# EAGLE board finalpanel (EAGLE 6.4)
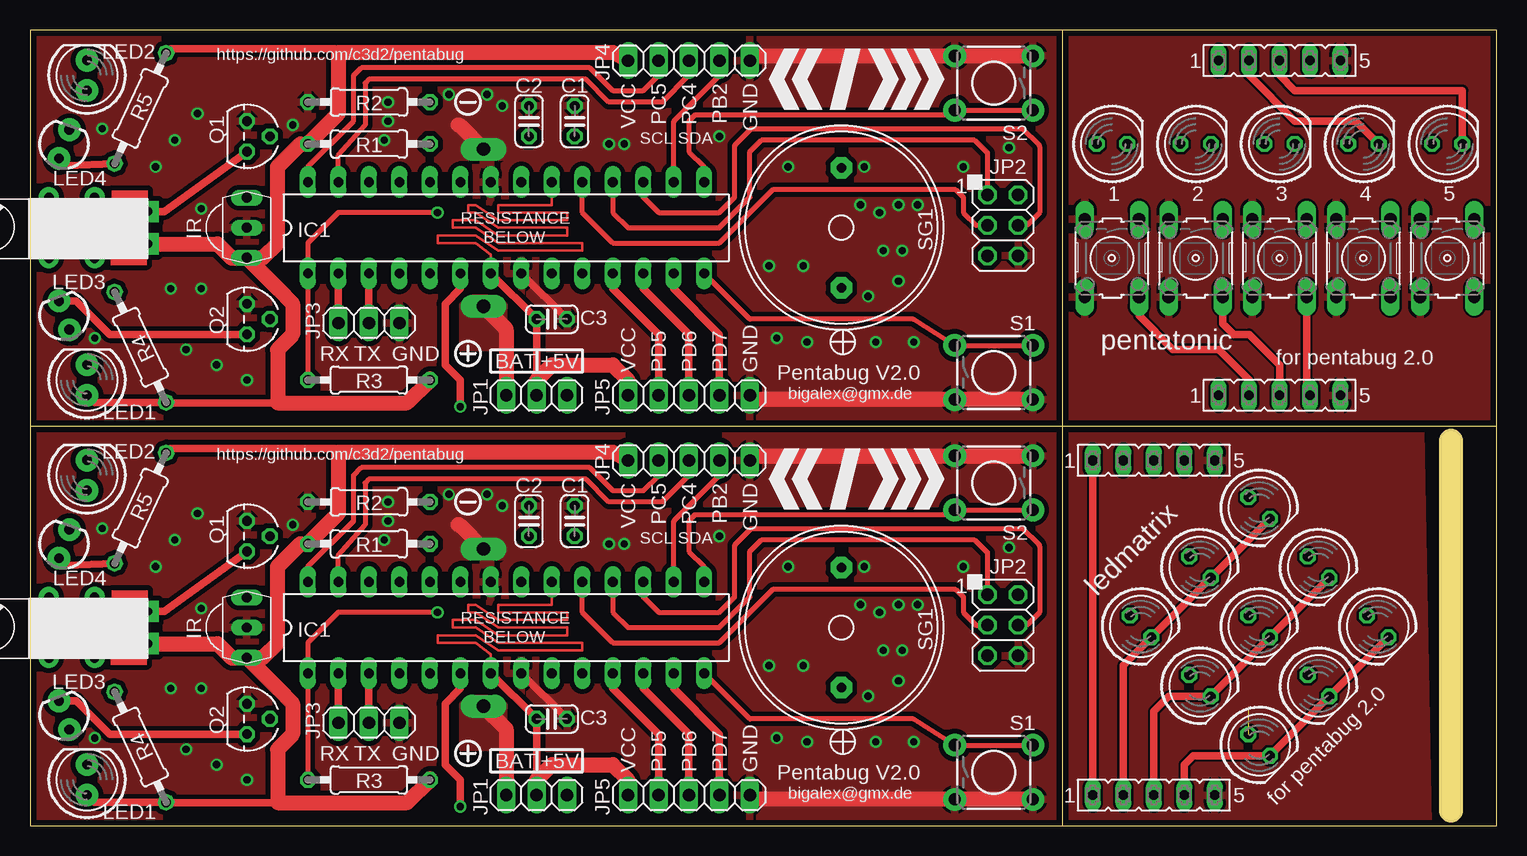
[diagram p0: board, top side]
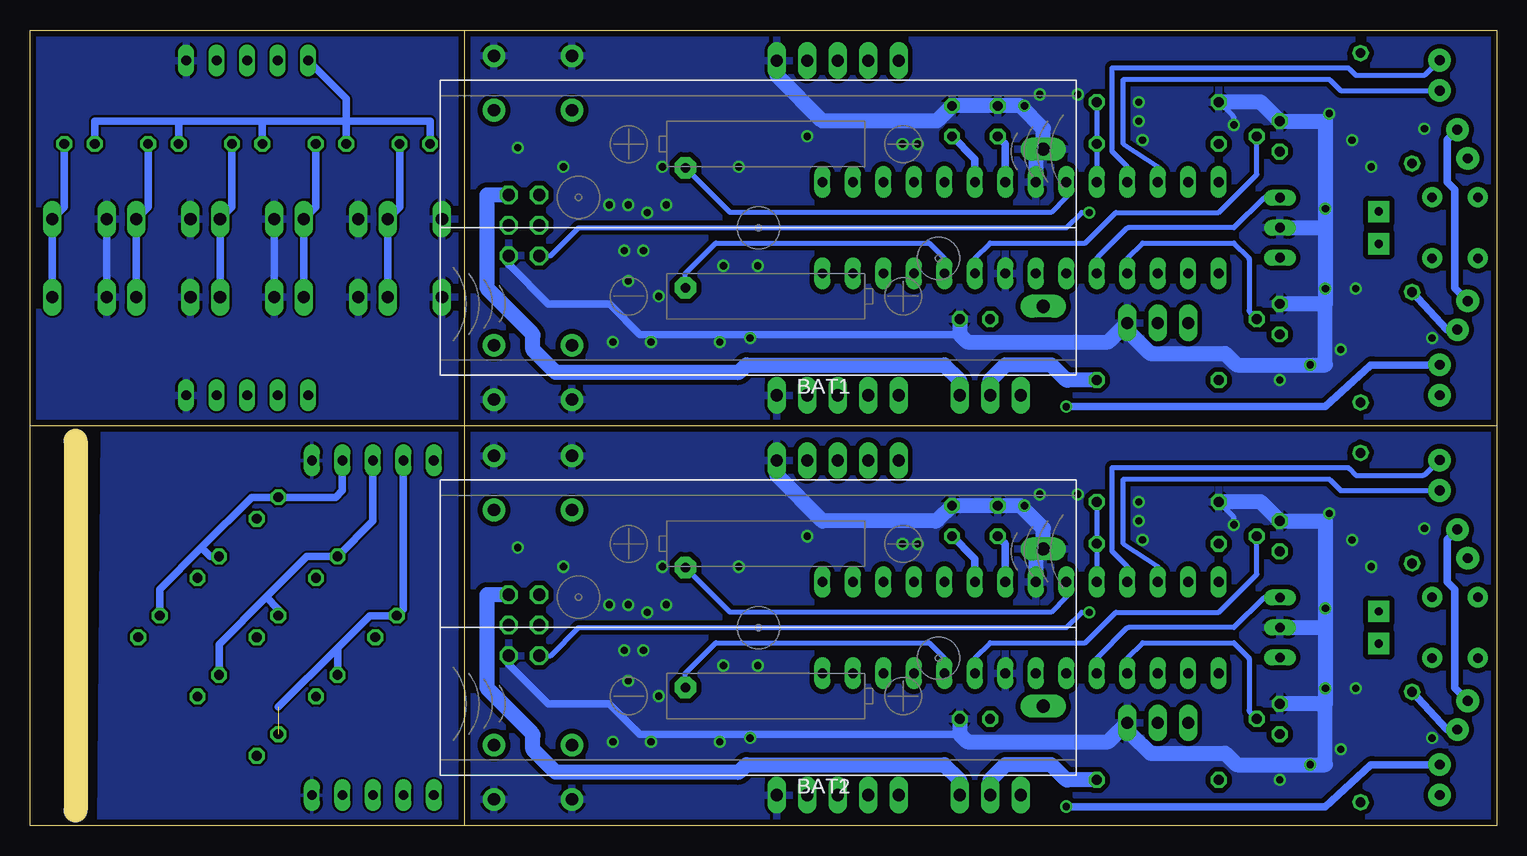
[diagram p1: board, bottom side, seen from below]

Size 122.22 x 66.34 mm. Coordinates in mm from the lower left corner, seen from the top.
Outline: 86.03,66.34 122.22,66.34 122.22,33.34
Outline: 86.03,66.34 86.03,0
Outline: 122.22,33.34 122.22,0 86.03,0
Outline: 86.03,66.34 0,66.34 0,33.34
Outline: 0,33.34 0,0 86.03,0
Outline: 0,33.34 122.22,33.34
Outline: 118.41,32.07 118.41,1.27
Copper layers (1*16): Top 0.035mm / dielectric 1.5mm / Bottom 0.035mm
Design rules "default *": minimum track width 8mil, minimum drill 0.6mm, track to track 8mil, track to pad 8mil, pad to pad 8mil, via to via 8mil, smd to smd 8mil, copper to edge 0.5mm, drill to drill 8mil, minimum pad ring 10mil, minimum via ring 8mil, stop-mask expansion 4mil, vias tented up to drill 0.8mm, thermal gap 10mil

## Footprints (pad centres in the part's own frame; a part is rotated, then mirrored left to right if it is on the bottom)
BATTERY_2XAAA_SMALLPINS = drill 1.1 pad 1.905 long: + -23.75,6.55; - -23.75,-6.55
C025-024X044 = drill 0.813 octagon: 1 -1.27,0; 2 1.27,0
DIL28-3 = drill 0.813 long: 1 -16.51,-3.81; 2 -13.97,-3.81; 3 -11.43,-3.81; 4 -8.89,-3.81; 5 -6.35,-3.81; 6 -3.81,-3.81; 7 -1.27,-3.81; 8 1.27,-3.81; 9 3.81,-3.81; 10 6.35,-3.81; 11 8.89,-3.81; 12 11.43,-3.81; 13 13.97,-3.81; 14 16.51,-3.81; 15 16.51,3.81; 16 13.97,3.81; 17 11.43,3.81; 18 8.89,3.81; 19 6.35,3.81; 20 3.81,3.81; 21 1.27,3.81; 22 -1.27,3.81; 23 -3.81,3.81; 24 -6.35,3.81; 25 -8.89,3.81; 26 -11.43,3.81; 27 -13.97,3.81; 28 -16.51,3.81
TSOP382 = drill 0.813 long: GND -0.001,-0.027; OUT -2.501,-0.027; VCC 2.499,-0.027
1X03 = drill 1.016 long: 1 -2.54,0; 2 0,0; 3 2.54,0
2X03 = drill 1.016 octagon: 1 -2.54,-1.27; 2 -2.54,1.27; 3 0,-1.27; 4 0,1.27; 5 2.54,-1.27; 6 2.54,1.27
1X05 = drill 1.016 long: 1 -5.08,0; 2 -2.54,0; 3 0,0; 4 2.54,0; 5 5.08,0
LED5MM = drill 0.813 pad 1.88: A -1.27,0; K 1.27,0
LED3MM = drill 0.813 pad 1.88: A -1.27,0; K 1.27,0
LED5MM' = drill 0.813 octagon: A -1.27,0; K 1.27,0
TO-92 = drill 0.813 octagon: 1 -1.27,0; 2 0,1.905; 3 1.27,0
0207/10 = drill 0.813 octagon: 1 -5.08,0; 2 5.08,0
TACTILE-PTH = drill 1.016 pad 1.88: 1 -3.251,2.261; 2 3.251,2.261; 3 -3.251,-2.261; 4 3.251,-2.261
B3F-10XX = drill 1.016 long: 1 -3.251,2.261; 2 3.251,2.261; 3 -3.251,-2.261; 4 3.251,-2.261
BUZZRTDK = drill 0.8 pad 1.8 octagon: + 5,0; - -5,0
FE05-1 = drill 0.813 long: 1 -5.08,0; 2 -2.54,0; 3 0,0; 4 2.54,0; 5 5.08,0
LA4-432 = drill 0.7 pad 1.778 square: P$1 -6.985,1.35; P$2 -6.985,-1.35

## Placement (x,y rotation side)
BAT1  BATTERY_2XAAA  [BATTERY_2XAAA_SMALLPINS]  61.53,49.85 180 bottom
BAT2  BATTERY_2XAAA  [BATTERY_2XAAA_SMALLPINS]  61.53,16.51 180 bottom
C1  100nF  [C025-024X044]  45.39,58.74 270 top
C2  100nF  [C025-024X044]  41.58,58.74 270 top
C3  100nF  [C025-024X044]  43.48,42.23 180 top
C4  100nF  [C025-024X044]  45.39,25.4 270 top
C5  100nF  [C025-024X044]  41.58,25.4 270 top
C6  100nF  [C025-024X044]  43.48,8.89 180 top
IC1  ATMEGA88  [DIL28-3]  39.67,49.85 0 top
IC2  ATMEGA88  [DIL28-3]  39.67,16.51 0 top
IR  TSOP382  [TSOP382]  18.09,49.85 270 top
IR1  TSOP382  [TSOP382]  18.09,16.51 270 top
JP1  [1X03]  42.21,35.88 180 top
JP2  [2X03]  81.07,50.05 270 top
JP3  [1X03]  28.25,41.91 0 top
JP4  [1X05]  54.91,63.79 0 top
JP5  [1X05]  54.91,35.88 0 top
JP6  [1X03]  28.25,8.57 0 top
JP7  [2X03]  81.07,16.71 270 top
JP8  [1X05]  54.91,2.54 0 top
JP9  [1X05]  54.91,30.45 0 top
JP10  [1X03]  42.21,2.54 180 top
LED1  [LED5MM]  4.75,37.15 90 top
LED2  [LED5MM]  4.75,62.55 90 top
LED3  [LED3MM]  2.85,42.55 110 top
LED4  [LED3MM]  2.85,56.83 70 top
LED5  [LED5MM']  90.16,56.83 0 top
LED6  [LED5MM']  97.14,56.83 0 top
LED7  [LED5MM']  104.13,56.83 0 top
LED8  [LED5MM']  111.11,56.83 0 top
LED9  [LED5MM']  118.1,56.83 0 top
LED10  [LED5MM']  102.43,26.48 315 top
LED11  [LED5MM']  107.37,21.54 315 top
LED12  [LED5MM']  112.31,16.6 315 top
LED13  [LED5MM']  97.49,21.54 315 top
LED14  [LED5MM']  102.43,16.6 315 top
LED15  [LED5MM']  107.37,11.66 315 top
LED16  [LED5MM']  92.55,16.6 315 top
LED17  [LED5MM']  97.49,11.66 315 top
LED18  [LED5MM']  102.43,6.72 315 top
LED19  [LED5MM]  4.75,3.81 90 top
LED20  [LED5MM]  4.75,29.21 90 top
LED21  [LED3MM]  2.85,9.21 110 top
LED22  [LED3MM]  2.85,23.49 70 top
Q1  [TO-92]  18.09,57.47 270 top
Q2  [TO-92]  18.09,42.23 270 top
Q3  [TO-92]  18.09,24.13 270 top
Q4  [TO-92]  18.09,8.89 270 top
R1  100K  [0207/10]  28.25,56.83 0 top
R2  22K  [0207/10]  28.25,60.33 180 top
R3  10k  [0207/10]  28.25,37.15 0 top
R4  22R  [0207/10]  9.2,39.89 295 top
R5  22R  [0207/10]  9.2,59.81 65 top
R6  10k  [0207/10]  28.25,3.81 0 top
R7  100K  [0207/10]  28.25,23.49 0 top
R8  22K  [0207/10]  28.25,26.99 180 top
R9  22R  [0207/10]  9.2,6.55 295 top
R10  22R  [0207/10]  9.2,26.47 65 top
S1  [TACTILE-PTH]  80.31,37.78 0 top
S2  [TACTILE-PTH]  80.31,61.91 180 top
S3  [B3F-10XX]  90.16,47.31 270 top
S4  [B3F-10XX]  97.14,47.31 270 top
S5  [B3F-10XX]  104.13,47.31 270 top
S6  [B3F-10XX]  111.11,47.31 270 top
S7  [B3F-10XX]  118.1,47.31 270 top
S8  [TACTILE-PTH]  80.31,28.57 180 top
S9  [TACTILE-PTH]  80.31,4.45 0 top
SG1  MULTIBUZZRTDKBUZZR  [BUZZRTDK]  67.61,49.85 270 top
SG2  MULTIBUZZRTDKBUZZR  [BUZZRTDK]  67.61,16.51 270 top
SV4  [FE05-1]  104.13,35.88 0 top
SV5  [FE05-1]  104.13,63.79 0 top
SV__4  [FE05-1]  93.65,2.54 0 top
SV__5  [FE05-1]  93.65,30.45 0 top
U$1  VIBRAMOTOR  [LA4-432]  2.85,49.85 180 top
U$2  VIBRAMOTOR  [LA4-432]  2.85,16.51 180 top

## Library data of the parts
BAT1 BAT2 IR IR1 SG1 SG2 U$1 U$2 = buglbr
C1-C6 = resistor
IC1 IC2 = atmel; OC_FARNELL: unknown; OC_NEWARK: unknown
JP1-JP10 = pinhead
LED1-LED4 LED19-LED22 S1 S2 S8 S9 = SparkFun
LED5-LED18 = led
Q1-Q4 = transistors
R1-R10 = rcl
S3-S7 = switch-omron; MPN: B3F-1000; OC_FARNELL: 176432; OC_NEWARK: 36M3542
SV4 SV5 SV__4 SV__5 = con-lsta; OC_FARNELL: unknown; OC_NEWARK: unknown

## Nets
+5V: JP1.1 JP2.2
+5V1: JP7.2 JP10.1
BAT: BAT1.+ JP1.3
BAT1: BAT2.+ JP10.3
BATLVL: IC1.24 R1.2 R2.1
BATLVL1: IC2.24 R7.2 R8.1
BUZGND: IC1.23 SG1.-
BUZGND1: IC2.23 SG2.-
BUZZR: IC1.10 SG1.+
BUZZR1: IC2.10 SG2.+
GND: BAT1.- C1.1 C2.1 C3.1 IC1.8 IC1.22 IR.GND JP2.6 JP3.3 JP4.5 JP5.5 Q1.1 Q2.1 R2.2 S1.3 S1.4 S2.3 S2.4
GND1: BAT2.- C4.1 C5.1 C6.1 IC2.8 IC2.22 IR1.GND JP6.3 JP7.6 JP8.5 JP9.5 Q3.1 Q4.1 R8.2 S8.3 S8.4 S9.3 S9.4
GND_L: SV__4.5 SV__5.5
GND_M: S3.3 S3.4 S4.3 S4.4 S5.3 S5.4 S6.3 S6.4 S7.3 S7.4 SV4.5 SV5.5
IRREC: IC1.5 IR.OUT
IRREC1: IC2.5 IR1.OUT
IRSEND: IC1.4 Q2.2
IRSEND1: IC2.4 Q4.2
MISO: IC1.18 JP2.1
MISO1: IC2.18 JP7.1
MOSI: IC1.17 JP2.4
MOSI1: IC2.17 JP7.4
N$3: IC1.26 LED2.A
N$5: IC1.25 LED2.K
N$7: LED4.A R5.1
N$8: Q1.3 U$1.P$2
N$9: C5.2 IC2.21
N$10: LED3.A R4.1
N$11: LED3.K LED4.K Q2.3
N$12: IC1.6 LED1.K
N$13: Q3.3 U$2.P$2
N$17: C2.2 IC1.21
N$19: IC2.26 LED20.A
N$20: IC2.25 LED20.K
N$21: LED22.A R10.1
N$22: LED21.A R9.1
N$23: LED21.K LED22.K Q4.3
N$24: IC2.6 LED19.K
PB1: IC2.16 JP9.4
PB2: IC1.16 JP4.4
PB2_L: LED12.K LED15.K LED18.K SV__4.4
PB2_T: LED7.K S5.1 S5.2 SV4.4
PC4_L: LED11.K LED14.K LED17.K SV__4.3
PC4_T: LED6.K S4.1 S4.2 SV4.3
PC5_L: LED10.K LED13.K LED16.K SV__4.2
PC5_T: LED5.K S3.1 S3.2 SV4.2
PD1: IC2.11 JP8.2
PD2: IC2.12 JP8.3
PD3: IC2.13 JP8.4
PD5: IC1.11 JP5.2
PD5_L: LED16.A LED17.A LED18.A SV__5.2
PD5_T: LED8.K S6.1 S6.2 SV5.2
PD6: IC1.12 JP5.3
PD6_L: LED13.A LED14.A LED15.A SV__5.3
PD6_T: LED9.K S7.1 S7.2 SV5.3
PD7: IC1.13 JP5.4
PD7_L: LED10.A LED11.A LED12.A SV__5.4
RST: IC1.1 JP2.5 R3.1
RST1: IC2.1 JP7.5 R6.1
RX: IC1.2 JP3.1
RX1: IC2.2 JP6.1
S1: IC1.14 S1.1 S1.2
S2: IC1.15 S2.1 S2.2
S3: IC2.14 S9.1 S9.2
S4: IC2.15 S8.1 S8.2
SCK: IC1.19 JP2.3
SCK1: IC2.19 JP7.3
SCL: IC1.28 JP4.2
SCL1: IC2.28 JP9.2
SDA: IC1.27 JP4.3
SDA1: IC2.27 JP9.3
TX: IC1.3 JP3.2
TX1: IC2.3 JP6.2
VCC: C1.2 C3.2 IC1.7 IC1.20 IR.VCC JP1.2 JP4.1 JP5.1 LED1.A R1.1 R3.2 R4.2 R5.2 U$1.P$1
VCC1: C4.2 C6.2 IC2.7 IC2.20 IR1.VCC JP8.1 JP9.1 JP10.2 LED19.A R6.2 R7.1 R9.2 R10.2 U$2.P$1
VCC_L: SV__4.1 SV__5.1
VCC_M: LED5.A LED6.A LED7.A LED8.A LED9.A SV5.1
VIBRATE: IC1.9 Q1.2
VIBRATE1: IC2.9 Q3.2

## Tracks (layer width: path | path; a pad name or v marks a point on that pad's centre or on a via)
+5V
  Bottom 1.27: JP2.2 84.12,52.59 84.12,44.87 arc-45 84.05,44.69 80.39,41.03 arc45 80.31,40.85 80.31,39.69 78.48,37.86 arc-45 78.3,37.78 63.27,37.78 arc-45 63.1,37.86 62.53,38.42 46.02,38.42 44.83,37.22 arc45 44.75,37.04 JP1.1
+5V1
  Bottom 1.27: JP7.2 84.12,19.25 84.12,11.54 arc-45 84.05,11.36 80.39,7.69 arc45 80.31,7.51 80.31,6.35 78.48,4.52 arc-45 78.3,4.45 63.27,4.45 arc-45 63.1,4.52 62.53,5.08 46.02,5.08 44.83,3.88 arc45 44.75,3.7 JP10.1
BAT
  Top 1.27: BAT1.+ 39.6,41.48 arc-45 39.67,41.3 JP1.3
  pour Top (no thermals): 36.82,44.13 35.86,43.5 35.86,39.69 39.67,39.69 39.67,43.5 38.09,44.13
BAT1
  Top 1.27: BAT2.+ 39.6,8.14 arc-45 39.67,7.96 JP10.3
  pour Top (no thermals): 36.82,10.79 35.86,10.16 35.86,6.35 39.67,6.35 39.67,10.16 38.09,10.79
BATLVL
  Bottom 0.406: R2.1 R1.2 IC1.24
BATLVL1
  Bottom 0.406: R8.1 R7.2 IC2.24
BUZGND
  Bottom 0.406: IC1.23 35.86,52.39 37.13,51.12 63.88,51.12 SG1.-
BUZGND1
  Bottom 0.406: IC2.23 35.86,19.05 37.13,17.78 63.88,17.78 SG2.-
BUZZR
  Bottom 0.406: SG1.+ 67.61,46.04 65.08,48.58 47.29,48.58 46.02,47.31 IC1.10
BUZZR1
  Bottom 0.406: SG2.+ 67.61,12.7 65.08,15.24 47.29,15.24 46.02,13.97 IC2.10
GND  (via drill 0.6)
  Top 0.61: IC1.8 C3.1
  Top 1.27: 35.66,58.42 arc-45 35.84,58.35 BAT1.- | JP4.5 60.31,64.1 arc-45 60.49,64.17 S2.4 S2.3 | S1.4 S1.3 60.46,35.52 arc-45 60.28,35.6 JP5.5
  Bottom 0.406: v21.89,58.42 21.89,58.95 arc-45 21.97,59.13 R2.2
  Bottom 0.61: 44.75,40.96 71.42,40.96 73.89,43.42 arc-45 74.07,43.5 79.05,43.5 82.26,46.72 arc45 82.34,46.9 JP2.6
  Bottom 1.27: IC1.22 38.4,55.78 BAT1.- 37.78,58.12 39.67,60.01 C2.1 C1.1 46.59,58.81 arc45 46.76,58.74 56.18,58.74 59.92,62.47 arc45 59.99,62.65 JP4.5 | 14.28,49.85 14.28,58.74 Q1.1 19.67,60.33 R2.2 | 14.28,49.85 14.28,43.5 | 14.28,43.5 Q2.1 | IR.GND 14.28,49.85 | C3.1 44.75,40.96 44.19,40.4 arc-45 44.01,40.32 32.48,40.32 arc-45 32.3,40.4 JP3.3 30.79,40.96 30.57,40.96 arc45 30.39,40.88 28.88,39.37 22.64,39.37 21.76,38.49 arc-45 21.58,38.42 14.28,38.42 14.28,43.5
  other vias: 29.83,58.74 29.83,60.33 29.52,57.15 34.91,60.96 57.45,57.47 38.09,60.96 39.36,60.01 48.25,56.83 49.52,56.83 63.17,54.93 69.52,54.93 81.58,56.52 77.77,54.93 73.97,51.75 72.38,51.75 70.79,51.12 69.2,51.75 72.69,47.94 71.11,47.94 64.44,46.67 61.58,46.67 72.38,45.4 69.84,44.13 62.22,40.64 64.76,40.32 70.47,40.32 73.65,40.32 18.09,37.15 15.55,38.42 13.01,39.69 11.73,44.77 14.28,44.77 14.28,51.44 10.46,54.93 12.05,57.15 13.96,59.37 6.02,58.1 5.38,40.64
  pour Top (isolate 0.406): -0.96,33.34 -0.96,67.63 86.03,67.63 86.03,33.34
  pour Bottom (isolate 0.406): -0.96,33.34 -0.96,67.63 86.03,67.94 86.03,33.66
  pour Top (no thermals): 35.55,55.56 39.99,55.56 39.99,57.47 38.4,58.74 35.55,58.74
GND1  (via drill 0.6)
  Top 0.61: IC2.8 C6.1
  Top 1.27: 35.66,25.08 arc-45 35.84,25.01 BAT2.- | JP9.5 60.31,30.76 arc-45 60.49,30.84 S8.4 S8.3 | S9.4 S9.3 60.46,2.18 arc-45 60.28,2.26 JP8.5
  Bottom 0.406: v21.89,25.08 21.89,25.61 arc-45 21.97,25.79 R8.2
  Bottom 0.61: 44.75,7.62 71.42,7.62 73.89,10.09 arc-45 74.07,10.16 79.05,10.16 82.26,13.38 arc45 82.34,13.56 JP7.6
  Bottom 1.27: IC2.22 38.4,22.44 BAT2.- 37.78,24.78 39.67,26.67 C5.1 C4.1 46.59,25.47 arc45 46.76,25.4 56.18,25.4 59.92,29.14 arc45 59.99,29.32 JP9.5 | 14.28,16.51 14.28,25.4 Q3.1 19.67,26.99 R8.2 | 14.28,16.51 14.28,10.16 | 14.28,10.16 Q4.1 | IR1.GND 14.28,16.51 | C6.1 44.75,7.62 44.19,7.06 arc-45 44.01,6.99 32.48,6.99 arc-45 32.3,7.06 JP6.3 30.79,7.62 30.57,7.62 arc45 30.39,7.55 28.88,6.03 22.64,6.03 21.76,5.15 arc-45 21.58,5.08 14.28,5.08 14.28,10.16
  other vias: 29.83,25.4 29.83,26.99 29.52,23.81 34.91,27.62 57.45,24.13 38.09,27.62 39.36,26.67 48.25,23.49 49.52,23.49 63.17,21.59 69.52,21.59 81.58,23.18 77.77,21.59 73.97,18.41 72.38,18.41 70.79,17.78 69.2,18.41 72.69,14.6 71.11,14.6 64.44,13.33 61.58,13.33 72.38,12.06 69.84,10.79 62.22,7.3 64.76,6.98 70.47,6.98 73.65,6.98 18.09,3.81 15.55,5.08 13.01,6.35 11.73,11.43 14.28,11.43 14.28,18.1 10.46,21.59 12.05,23.81 13.96,26.03 6.02,24.77 5.38,7.3
  pour Top (isolate 0.406): -0.96,0 -0.96,33.34 86.03,33.34 86.03,0
  pour Bottom (isolate 0.406): -0.96,0 -0.96,33.34 86.03,33.34 86.03,0.32
  pour Top (no thermals): 35.55,22.22 39.99,22.22 39.99,24.13 38.4,25.4 35.55,25.4
GND_L
  pour Top: 85.39,33.02 115.88,33.02 116.51,0 86.03,0
  pour Bottom: 85.71,33.02 116.19,33.02 116.51,0 86.03,0
GND_M
  Bottom 0.61: S5.3 S5.4 | S7.3 S7.4
  pour Top: 86.35,33.34 121.91,33.34 121.91,66.36 86.35,66.36
  pour Bottom: 86.35,66.36 121.91,66.36 121.91,33.34 86.35,33.34
IRREC
  Bottom 0.406: IC1.5 33.32,47.2 arc45 33.25,47.38 30.86,49.77 arc45 30.68,49.85 21.89,49.85 19.47,52.27 arc45 19.29,52.35 IR.OUT
IRREC1
  Bottom 0.406: IC2.5 33.32,13.86 arc45 33.25,14.04 30.86,16.44 arc45 30.68,16.51 21.89,16.51 19.47,18.94 arc45 19.29,19.01 IR1.OUT
IRSEND
  Bottom 0.406: IC1.4 30.79,47.31 29.52,48.58 21.89,48.58 20.7,47.38 arc45 20.62,47.2 20.62,42.97 arc-45 20.55,42.79 Q2.2
IRSEND1
  Bottom 0.406: IC2.4 30.79,13.97 29.52,15.24 21.89,15.24 20.7,14.04 arc45 20.62,13.86 20.62,9.63 arc-45 20.55,9.45 Q4.2
MISO
  Top 0.406: IC1.18 48.56,51.12 49.83,49.85 57.45,49.85 59.99,52.39 59.99,56.2 60.95,57.15 78.73,57.15 79.8,56.08 JP2.1
MISO1
  Top 0.406: IC2.18 48.56,17.78 49.83,16.51 57.45,16.51 59.99,19.05 59.99,22.86 60.95,23.81 78.73,23.81 79.8,22.74 JP7.1
MOSI
  Top 0.406: IC1.17 51.1,52.39 52.38,51.12 57.45,51.12 58.65,52.31 arc45 58.72,52.49 58.72,56.62 arc-45 58.8,56.8 60.1,58.1 82.75,58.1 84.05,56.8 arc-45 84.12,56.62 84.12,51.12 83.13,50.12 arc-45 82.95,50.05 JP2.4
MOSI1
  Top 0.406: IC2.17 51.1,19.05 52.38,17.78 57.45,17.78 58.65,18.98 arc45 58.72,19.16 58.72,23.28 arc-45 58.8,23.46 60.1,24.77 82.75,24.77 84.05,23.46 arc-45 84.12,23.28 84.12,17.78 83.13,16.78 arc-45 82.95,16.71 JP7.4
N$1  (via drill 0.8 pad 1.68)
  other vias: 1.58,52.39
N$2  (via drill 0.8 pad 1.68)
  other vias: 5.38,52.39
N$3
  Bottom 0.406: IC1.26 28.25,54.93 31.1,56.83 31.1,62.23 14.06,62.23 arc45 13.88,62.16 13.01,61.28 LED2.A
N$4  (via drill 0.8 pad 1.68)
  other vias: 5.38,47.31
N$5
  Bottom 0.406: IC1.25 30.79,54.93 32.05,56.2 32.05,63.18 12.47,63.18 arc45 12.3,63.11 11.73,62.55 6.12,62.55 arc-45 5.95,62.62 LED2.K
N$6  (via drill 0.8 pad 1.68)
  other vias: 1.58,47.31
N$7
  Top 0.61: R5.1 3.02,55.03 arc-90 LED4.A
N$8
  Top 0.61: U$1.P$2 11.18,51.2 Q1.3
N$9
  Bottom 0.61: C5.2 41.02,23.57 arc45 40.94,23.39 IC2.21
N$10
  Bottom 0.61: LED3.A 4.15,41.35 R4.1
N$11
  Top 0.61: LED3.K 3.87,43.74 6.66,40.96 Q2.3
  Bottom 0.61: LED4.K 4.12,57.19 4.12,53.66 3.48,53.02 3.48,44.81 LED3.K
N$12  (via drill 0.6)
  Top 0.61: IC1.6 35.86,44.77 34.59,43.5 34.59,38.42 35.79,37.22 arc-45 35.86,37.04 v35.86,34.92
  Bottom 0.61: v35.86,34.92 14.28,34.92 10.54,38.34 arc45 10.36,38.42 LED1.K
N$13
  Top 0.61: U$2.P$2 11.18,17.86 Q3.3
N$14  (via drill 0.8 pad 1.68)
  other vias: 1.58,19.05
N$15  (via drill 0.8 pad 1.68)
  other vias: 5.38,19.05
N$16  (via drill 0.8 pad 1.68)
  other vias: 5.38,13.97
N$17
  Bottom 0.61: C2.2 41.02,56.91 arc45 40.94,56.73 IC1.21
N$18  (via drill 0.8 pad 1.68)
  other vias: 1.58,13.97
N$19
  Bottom 0.406: IC2.26 28.25,21.59 31.1,23.5 31.1,28.89 14.06,28.89 arc45 13.88,28.82 13.01,27.94 LED20.A
N$20
  Bottom 0.406: IC2.25 30.79,21.59 32.05,22.86 32.05,29.84 12.47,29.84 arc45 12.3,29.77 11.73,29.21 6.12,29.21 arc-45 5.95,29.28 LED20.K
N$21
  Top 0.61: R10.1 3.02,21.7 arc-90 LED22.A
N$22
  Bottom 0.61: LED21.A 4.15,8.01 R9.1
N$23
  Top 0.61: LED21.K 3.87,10.4 6.66,7.62 Q4.3
  Bottom 0.61: LED22.K 4.12,23.85 4.12,20.32 3.48,19.69 3.48,11.47 LED21.K
N$24  (via drill 0.6)
  Top 0.61: IC2.6 35.86,11.43 34.59,10.16 34.59,5.08 35.79,3.88 arc-45 35.86,3.7 v35.86,1.59
  Bottom 0.61: v35.86,1.59 14.28,1.59 10.54,5.01 arc45 10.36,5.08 LED19.K
PB1
  Top 0.406: IC2.16 53.64,25.29 arc-45 53.72,25.47 57.38,29.14 arc45 57.45,29.32 JP9.4
PB2
  Top 0.406: IC1.16 53.64,58.63 arc-45 53.72,58.81 57.38,62.47 arc45 57.45,62.65 JP4.4
PB2_L
  Top 0.61: LED12.K LED15.K LED18.K 96.93,5.82 96.19,5.08 SV__4.4
PB2_T
  Top 0.61: SV4.4 106.39,35.88 S5.2
  Bottom 0.61: LED7.K 105.4,51.55 S5.1 S5.2
PC4_L
  Top 0.61: LED11.K LED14.K LED17.K 94.89,10.76 93.65,9.53 SV__4.3
PC4_T
  Top 0.61: S4.2 99.4,41.87 100.32,40.96 101.59,40.96 104.13,38.42 SV4.3
  Bottom 0.61: LED6.K 98.41,51.55 S4.1 S4.2
PC5_L
  Top 0.61: SV__4.2 91.11,13.36 92.68,14.94 LED16.K | LED16.K LED10.K | LED13.K LED16.K
PC5_T
  Top 0.61: SV4.2 101.59,37.15 99.05,39.69 95.24,39.69 92.42,42.51 S3.2
  Bottom 0.61: LED5.K 91.43,51.55 S3.1 S3.2
PD1
  Top 0.61: IC2.11 48.56,11.43 52.38,7.62 JP8.2
PD2
  Top 0.61: IC2.12 51.1,11.43 54.84,7.69 arc-45 54.91,7.51 JP8.3
PD3
  Top 0.61: IC2.13 53.64,11.43 57.45,7.62 JP8.4
PD5
  Top 0.61: IC1.11 48.56,44.77 52.38,40.96 JP5.2
PD5_L  (1 unrouted)
  Bottom 0.61: SV__5.2 91.11,18.04 LED16.A 93.93,17.5 96.59,14.84 | 96.59,14.84 101.53,9.9 | LED17.A 96.59,14.84
PD5_T
  Top 0.61: SV5.2 101.59,62.55 105.4,58.74 110.48,58.74 LED8.K
  Bottom 0.61: LED8.K 112.38,51.55 S6.1 S6.2
PD6
  Top 0.61: IC1.12 51.1,44.77 54.84,41.03 arc-45 54.91,40.85 JP5.3
PD6_L
  Bottom 0.61: 102.54,19.05 99.15,22.44 LED13.A 96.59,22.46 93.65,25.4 SV__5.3 | 102.54,19.05 106.47,15.12 LED15.A | LED14.A 101.53,18.04 102.54,19.05
PD6_T
  Top 0.61: LED9.K 119.37,61.28 105.4,61.28 104.13,62.55 SV5.3
  Bottom 0.61: LED9.K 119.37,51.55 S7.1 | S7.1 120.36,50.84 120.64,51.12 | S7.1 S7.2
PD7
  Top 0.61: IC1.13 53.64,44.77 57.45,40.96 JP5.4
PD7_L
  Bottom 0.61: 107.94,23.18 111.41,19.7 LED12.A | LED11.A 107.2,22.44 107.94,23.18 | 107.94,23.18 103.74,27.38 LED10.A 96.75,27.38 96.19,27.94 SV__5.4
RST  (via drill 0.6)
  Top 0.406: v33.96,51.12 25.71,51.12 23.16,48.58 IC1.1 R3.1
  Bottom 0.406: JP2.5 78.84,47.51 76.5,49.85 35.86,49.85 34.59,51.12 v33.96,51.12
RST1  (via drill 0.6)
  Top 0.406: v33.96,17.78 25.71,17.78 23.16,15.24 IC2.1 R6.1
  Bottom 0.406: JP7.5 78.84,14.17 76.5,16.51 35.86,16.51 34.59,17.78 v33.96,17.78
RX
  Top 0.61: JP3.1 IC1.2
RX1
  Top 0.61: JP6.1 IC2.2
S1
  Top 0.406: S1.2 S1.1 73.61,42.23 59.99,42.23 IC1.14
S2
  Top 0.406: S2.1 S2.2 76.67,59.26 55.44,59.26 54.91,58.74 54.91,56.2 56.18,54.93 IC1.15
S3
  Top 0.406: S9.2 S9.1 73.61,8.89 59.99,8.89 IC2.14
S4
  Top 0.406: S8.1 S8.2 76.67,25.92 55.44,25.92 54.91,25.4 54.91,22.86 56.18,21.59 IC2.15
SCK
  Top 0.406: IC1.19 46.02,51.12 48.56,48.58 57.45,48.58 61.9,53.02 77.14,53.02 77.77,52.39 77.77,51.12 78.84,50.05 JP2.3
SCK1
  Top 0.406: IC2.19 46.02,17.78 48.56,15.24 57.45,15.24 61.9,19.69 77.14,19.69 77.77,19.05 77.77,17.78 78.84,16.71 JP7.3
SCL
  Top 0.406: JP4.2 52.38,62.55 51.1,61.28 48.56,61.28 46.66,63.18 27.61,63.18 26.98,62.55 26.98,58.74 23.16,54.93 IC1.28
SCL1
  Top 0.406: JP9.2 52.38,29.21 51.1,27.94 48.56,27.94 46.66,29.84 27.61,29.84 26.98,29.21 26.98,25.4 23.16,21.59 IC2.28
SDA
  Top 0.406: JP4.3 54.91,62.55 52.69,60.33 48.25,60.33 46.34,62.23 28.25,62.23 27.93,61.91 27.93,58.42 25.71,55.88 IC1.27
SDA1
  Top 0.406: JP9.3 54.91,29.21 52.69,26.99 48.25,26.99 46.34,28.89 28.25,28.89 27.93,28.57 27.93,25.08 25.71,22.54 IC2.27
TX
  Top 0.61: JP3.2 IC1.3
TX1
  Top 0.61: JP6.2 IC2.3
VCC
  Top 0.203: IC1.7 38.4,47.62 37.13,48.58 33.96,48.58 33.96,49.21 37.13,49.21 39.04,47.94 46.02,47.94 46.02,48.58 39.04,48.58 37.13,49.85 35.23,49.85 35.23,50.48 37.13,50.48 39.04,49.21 44.75,49.21 44.75,49.85 39.04,49.85 37.13,51.12 36.5,51.12 36.5,51.75 37.13,51.75 39.04,50.48 44.75,50.48 44.75,51.12 39.04,51.12 39.04,51.75 43.48,51.75 IC1.20
  Top 0.61: IC1.7 C3.2 42.21,37.15 | 25.71,64.45 25.39,64.77 11.73,64.77 11.23,64.58 R5.2 | LED1.A 5.27,35.36 arc45 5.45,35.28 R4.2 arc45 11.44,35.24 20.62,35.24
  Top 1.27: JP4.1 48.56,64.45 25.71,64.45 25.71,59.37 R1.1 22.53,56.83 20.62,54.93 20.62,48.58 19.4,47.35 IR.VCC | U$1.P$1 15.62,48.5 16.82,47.31 18.02,47.31 IR.VCC | JP5.1 49.83,37.15 48.56,38.42 43.48,38.42 42.21,37.15 JP1.2 | IR.VCC 20.62,44.78 20.62,44.77 21.89,43.5 21.89,40.96 20.62,39.69 20.62,35.24 31.32,35.24 arc45 31.49,35.32 33.25,37.07 arc45 33.32,37.25 R3.2
  Bottom 0.61: IC1.20 43.48,55.46 arc-45 43.56,55.64 C1.2
  Bottom 1.27: 42.21,37.15 JP1.2 42.21,37.04 arc45 42.14,37.22 40.94,38.42 37.13,38.42 35.94,37.22 arc-45 35.76,37.15 R3.2
VCC1
  Top 0.203: IC2.7 38.4,14.29 37.13,15.24 33.96,15.24 33.96,15.88 37.13,15.88 39.04,14.6 46.02,14.6 46.02,15.24 39.04,15.24 37.13,16.51 35.23,16.51 35.23,17.15 37.13,17.15 39.04,15.88 44.75,15.88 44.75,16.51 39.04,16.51 37.13,17.78 36.5,17.78 36.5,18.42 37.13,18.42 39.04,17.15 44.75,17.15 44.75,17.78 39.04,17.78 39.04,18.42 43.48,18.42 IC2.20
  Top 0.61: IC2.7 C6.2 42.21,3.81 | 25.71,31.11 25.39,31.43 11.73,31.43 11.23,31.24 R10.2 | LED19.A 5.27,2.02 arc45 5.45,1.95 R9.2 arc45 11.44,1.9 20.62,1.9
  Top 1.27: JP9.1 48.56,31.11 25.71,31.11 25.71,26.03 R7.1 22.53,23.5 20.62,21.59 20.62,15.24 19.4,14.01 IR1.VCC | U$2.P$1 15.62,15.16 16.82,13.97 18.02,13.97 IR1.VCC | JP8.1 49.83,3.81 48.56,5.08 43.48,5.08 42.21,3.81 JP10.2 | IR1.VCC 20.62,11.44 20.62,11.43 21.89,10.16 21.89,7.62 20.62,6.35 20.62,1.9 31.32,1.9 arc45 31.49,1.98 33.25,3.74 arc45 33.32,3.92 R6.2
  Bottom 0.61: IC2.20 43.48,22.12 arc-45 43.56,22.3 C4.2
  Bottom 1.27: 42.21,3.81 JP10.2 42.21,3.7 arc45 42.14,3.88 40.94,5.08 37.13,5.08 35.94,3.88 arc-45 35.76,3.81 R6.2
VCC_L
  Top 0.61: SV__5.1 SV__4.1
VCC_M
  Bottom 0.61: SV5.1 95.87,60.61 95.87,58.74 | LED5.A 88.89,58.74 95.87,58.74 | LED6.A 95.87,58.74 | 95.87,58.74 102.86,58.74 | 102.86,58.74 109.84,58.74 | 109.84,58.74 116.83,58.74 LED9.A | LED7.A 102.86,58.74 | LED8.A 109.84,58.74
VIBRATE
  Bottom 0.406: IC1.9 43.48,47.31 42.21,48.58 34.28,48.58 31.74,51.12 23.16,51.12 19.99,54.29 Q1.2
VIBRATE1
  Bottom 0.406: IC2.9 43.48,13.97 42.21,15.24 34.28,15.24 31.74,17.78 23.16,17.78 19.99,20.95 Q3.2

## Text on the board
tNames: https://github.com/c3d2/pentabug | VCC | PC5 | PC4 | PB2 | GND | SCL | SDA | 1 | 1 | 2 | 3 | 4 | 5 | RESISTANCE | IR | BELOW | pentatonic | RX | TX | GND | BAT | +5V | for pentabug 2.0 | VCC | PD5 | PD6 | PD7 | GND | Pentabug V2.0 | bigalex@gmx.de | LED2 | https://github.com/c3d2/pentabug | JP4 | VCC | PC5 | PC4 | PB2 | GND | C2 | C1 | R2 | R5 | S2 | Q1 | SCL | SDA | R1 | JP2 | LED4 | 1 | ledmatrix | IC1 | RESISTANCE | IR | BELOW | SG1 | LED3 | S1 | C3 | Q2 | JP3 | R4 | RX | TX | GND | BAT | +5V | VCC | PD5 | PD6 | PD7 | GND | R3 | Pentabug V2.0 | bigalex@gmx.de | JP1 | JP5 | for pentabug 2.0 | LED1
_bNames: BAT1 | BAT1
